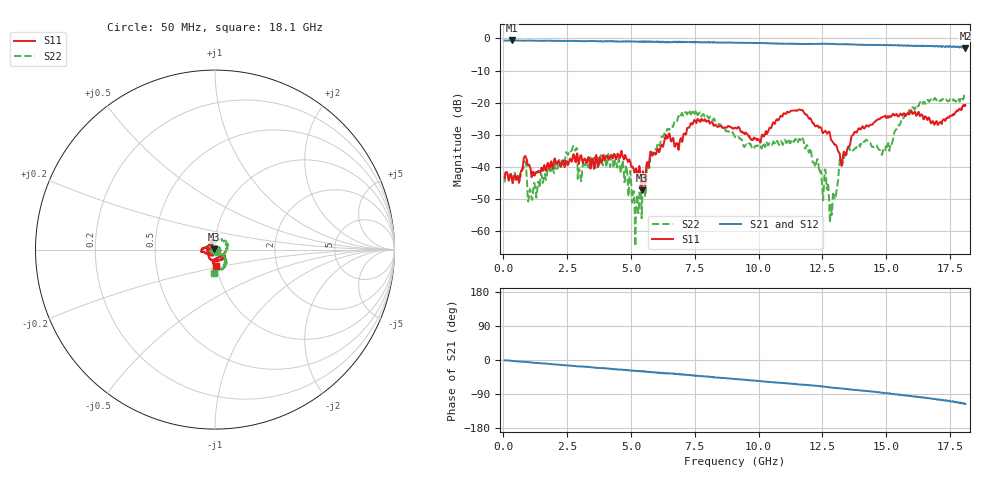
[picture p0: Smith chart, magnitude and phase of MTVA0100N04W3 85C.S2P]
! Network Analyzer HP8720D.06.14 Serial No. US36140669
! 17 Jan 2005  10:50:07
! Frequency  S11  S21  S12  S22
# HZ  S  DB R 50
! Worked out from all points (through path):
!   801 points, 50 MHz to 18.1 GHz, reference 50 ohm
!   highest |S21| = -0.63 dB at 343.3 MHz (marker M1); lowest = -2.9 dB at 18.1 GHz (marker M2)
!   group delay of S21, straight-line fit = 16.7 ps
!   lowest |S11| = -47.2 dB at 5.42 GHz (marker M3), VSWR 1.01, Z = 49.6 + j0.112 ohm
!   |S11| at or under -10 dB: start of sweep to end of sweep
!   |S22| runs from -64.6 to -17.4 dB; largest |S21 - S12| = 0.028
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5e7  -43.37 -18.9  -0.66 -0.9  -0.66 -1.1  -44.75 -9.0
3.433125e8  -43.93 -10.6  -0.63 -2.4  -0.65 -2.7  -44.13 -23.4
8.17125e8  -36.88 25.3  -0.70 -4.9  -0.69 -5.1  -39.69 -46.2
1.065312e9  -40.52 -8.8  -0.65 -6.3  -0.65 -6.5  -47.20 140.4
2.780062e9  -36.32 31.1  -0.76 -16.0  -0.76 -16.3  -34.10 110.5
3.073375e9  -37.18 65.0  -0.81 -17.2  -0.79 -17.5  -42.65 -113.3
4.607625e9  -35.32 50.7  -1.03 -25.1  -0.99 -25.5  -41.85 133.5
5.216812e9  -41.06 94.5  -0.98 -29.3  -1.00 -29.6  -50.69 135.4
5.419875e9  -47.21 165.0  -0.92 -30.4  -0.94 -30.5  -55.94 -145.4
6.074188e9  -34.52 -127.8  -1.10 -34.3  -1.11 -34.3  -32.64 132.8
7.337688e9  -26.46 108.1  -1.08 -40.4  -1.07 -40.4  -23.63 29.4
9.075e9  -27.84 -167.2  -1.35 -50.0  -1.32 -50.4  -30.52 -76.0
1.000006e10  -31.38 -164.7  -1.42 -55.4  -1.43 -55.6  -32.84 -78.1
1.166969e10  -22.27 -170.4  -1.68 -65.1  -1.69 -65.3  -32.12 -160.3
1.209838e10  -25.98 -152.1  -1.66 -67.2  -1.70 -67.5  -37.80 162.5
1.28655e10  -31.75 -107.5  -1.74 -72.7  -1.69 -73.3  -54.88 14.7
1.320394e10  -37.53 -118.7  -1.81 -74.8  -1.79 -75.1  -37.44 0.9
1.347469e10  -34.28 -118.1  -1.73 -76.8  -1.76 -76.8  -34.63 -39.0
1.509919e10  -24.57 -102.1  -2.16 -88.4  -2.04 -88.8  -34.34 -56.8
1.624988e10  -22.93 -36.4  -2.33 -96.8  -2.32 -97.6  -21.17 -50.7
1.708469e10  -26.18 -67.6  -2.48 -104.9  -2.38 -105.6  -19.23 -77.8
1.81e10  -20.77 -86.5  -2.93 -116.0  -2.86 -116.6  -17.55 -91.9
